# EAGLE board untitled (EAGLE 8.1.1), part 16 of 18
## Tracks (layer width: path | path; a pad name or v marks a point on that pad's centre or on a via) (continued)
S$16206 (continued)
  Bottom 0: 76.33,152.19 76.33,151.84
S$16207
  Bottom 0: 76.33,151.84 76.42,151.51
S$16208
  Bottom 0: 76.42,151.51 76.48,151.4
S$16209
  Bottom 0: 76.48,151.4 73.88,148.81
S$16210
  Bottom 0: 73.88,148.81 73.84,148.75
S$16211
  Bottom 0: 73.84,148.75 73.8,148.69
S$16212
  Bottom 0: 73.8,148.69 73.78,148.63
S$16213
  Bottom 0: 73.78,148.63 73.76,148.56
S$16214
  Bottom 0: 73.76,148.56 73.76,148.49
S$16215
  Bottom 0: 73.76,148.49 73.76,148.43
S$16216
  Bottom 0: 73.76,148.43 71.89,146.57
S$16217
  Bottom 0: 71.89,146.57 42.96,146.57
S$16218
  Bottom 0: 42.96,146.57 42.89,146.57
S$16219
  Bottom 0: 42.89,146.57 42.82,146.55
S$16220
  Bottom 0: 42.82,146.55 42.76,146.53
S$16221
  Bottom 0: 42.76,146.53 42.7,146.49
S$16222
  Bottom 0: 42.7,146.49 42.64,146.44
S$16223
  Bottom 0: 42.64,146.44 40.87,144.67
S$16224
  Bottom 0: 71.46,148.09 71.81,148.15
S$16225
  Bottom 0: 71.81,148.15 72.12,148.3
S$16226
  Bottom 0: 72.12,148.3 72.39,148.52
S$16227
  Bottom 0: 72.39,148.52 72.6,148.81
S$16228
  Bottom 0: 72.6,148.81 72.72,149.13
S$16229
  Bottom 0: 72.72,149.13 72.77,149.48
S$16230
  Bottom 0: 72.77,149.48 72.72,149.82
S$16231
  Bottom 0: 72.72,149.82 72.6,150.15
S$16232
  Bottom 0: 72.6,150.15 72.39,150.43
S$16233
  Bottom 0: 72.39,150.43 72.12,150.66
S$16234
  Bottom 0: 72.12,150.66 71.81,150.81
S$16235
  Bottom 0: 71.81,150.81 71.46,150.87
S$16236
  Bottom 0: 71.46,150.87 71.11,150.85
S$16237
  Bottom 0: 71.11,150.85 70.78,150.74
S$16238
  Bottom 0: 70.78,150.74 70.75,150.72
S$16239
  Bottom 0: 70.75,150.72 70.17,151.3
S$16240
  Bottom 0: 70.17,151.3 70.12,151.34
S$16241
  Bottom 0: 70.12,151.34 70.06,151.38
S$16242
  Bottom 0: 70.06,151.38 70,151.4
S$16243
  Bottom 0: 70,151.4 69.94,151.42
S$16244
  Bottom 0: 69.94,151.42 69.86,151.43
S$16245
  Bottom 0: 69.86,151.43 65.29,151.43
S$16246
  Bottom 0: 65.29,151.43 65.22,151.56
S$16247
  Bottom 0: 65.22,151.56 65.02,151.78
S$16248
  Bottom 0: 65.02,151.78 64.76,151.93
S$16249
  Bottom 0: 64.76,151.93 64.46,151.99
S$16250
  Bottom 0: 64.46,151.99 64.16,151.97
S$16251
  Bottom 0: 64.16,151.97 63.88,151.86
S$16252
  Bottom 0: 63.88,151.86 63.64,151.67
S$16253
  Bottom 0: 63.64,151.67 63.47,151.43
S$16254
  Bottom 0: 63.47,151.43 63.38,151.13
S$16255
  Bottom 0: 63.38,151.13 63.38,150.83
S$16256
  Bottom 0: 63.38,150.83 63.47,150.54
S$16257
  Bottom 0: 63.47,150.54 63.64,150.29
S$16258
  Bottom 0: 63.64,150.29 63.88,150.1
S$16259
  Bottom 0: 63.88,150.1 64.16,149.99
S$16260
  Bottom 0: 64.16,149.99 64.46,149.97
S$16261
  Bottom 0: 64.46,149.97 64.76,150.04
S$16262
  Bottom 0: 64.76,150.04 65.02,150.19
S$16263
  Bottom 0: 65.02,150.19 65.22,150.41
S$16264
  Bottom 0: 65.22,150.41 65.29,150.54
S$16265
  Bottom 0: 65.29,150.54 69.68,150.54
S$16266
  Bottom 0: 69.68,150.54 70.13,150.09
S$16267
  Bottom 0: 70.13,150.09 70.07,149.99
S$16268
  Bottom 0: 70.07,149.99 69.98,149.65
S$16269
  Bottom 0: 69.98,149.65 69.98,149.3
S$16270
  Bottom 0: 69.98,149.3 70.07,148.97
S$16271
  Bottom 0: 70.07,148.97 70.24,148.66
S$16272
  Bottom 0: 70.24,148.66 70.48,148.4
S$16273
  Bottom 0: 70.48,148.4 70.78,148.21
S$16274
  Bottom 0: 70.78,148.21 71.11,148.11
S$16275
  Bottom 0: 71.11,148.11 71.46,148.09
S$16276
  Bottom 0: 52.41,148.09 52.76,148.15
S$16277
  Bottom 0: 52.76,148.15 53.07,148.3
S$16278
  Bottom 0: 53.07,148.3 53.34,148.52
S$16279
  Bottom 0: 53.34,148.52 53.55,148.81
S$16280
  Bottom 0: 53.55,148.81 53.67,149.13
S$16281
  Bottom 0: 53.67,149.13 53.72,149.48
S$16282
  Bottom 0: 53.72,149.48 53.67,149.82
S$16283
  Bottom 0: 53.67,149.82 53.55,150.15
S$16284
  Bottom 0: 53.55,150.15 53.34,150.43
S$16285
  Bottom 0: 53.34,150.43 53.07,150.66
S$16286
  Bottom 0: 53.07,150.66 52.76,150.81
S$16287
  Bottom 0: 52.76,150.81 52.41,150.87
S$16288
  Bottom 0: 52.41,150.87 52.06,150.85
S$16289
  Bottom 0: 52.06,150.85 51.73,150.74
S$16290
  Bottom 0: 51.73,150.74 51.7,150.73
S$16291
  Bottom 0: 51.7,150.73 51.13,151.3
S$16292
  Bottom 0: 51.13,151.3 51.08,151.34
S$16293
  Bottom 0: 51.08,151.34 51.02,151.38
S$16294
  Bottom 0: 51.02,151.38 50.96,151.4
S$16295
  Bottom 0: 50.96,151.4 50.89,151.42
S$16296
  Bottom 0: 50.89,151.42 50.82,151.43
S$16297
  Bottom 0: 50.82,151.43 46.24,151.43
S$16298
  Bottom 0: 46.24,151.43 46.17,151.56
S$16299
  Bottom 0: 46.17,151.56 45.97,151.78
S$16300
  Bottom 0: 45.97,151.78 45.71,151.93
S$16301
  Bottom 0: 45.71,151.93 45.41,151.99
S$16302
  Bottom 0: 45.41,151.99 45.11,151.97
S$16303
  Bottom 0: 45.11,151.97 44.83,151.86
S$16304
  Bottom 0: 44.83,151.86 44.59,151.67
S$16305
  Bottom 0: 44.59,151.67 44.42,151.43
S$16306
  Bottom 0: 44.42,151.43 44.33,151.13
S$16307
  Bottom 0: 44.33,151.13 44.33,150.83
S$16308
  Bottom 0: 44.33,150.83 44.42,150.54
S$16309
  Bottom 0: 44.42,150.54 44.59,150.29
S$16310
  Bottom 0: 44.59,150.29 44.83,150.1
S$16311
  Bottom 0: 44.83,150.1 45.11,149.99
S$16312
  Bottom 0: 45.11,149.99 45.41,149.97
S$16313
  Bottom 0: 45.41,149.97 45.71,150.04
S$16314
  Bottom 0: 45.71,150.04 45.97,150.19
S$16315
  Bottom 0: 45.97,150.19 46.17,150.41
S$16316
  Bottom 0: 46.17,150.41 46.24,150.54
S$16317
  Bottom 0: 46.24,150.54 50.63,150.54
S$16318
  Bottom 0: 50.63,150.54 51.08,150.09
S$16319
  Bottom 0: 51.08,150.09 51.02,149.99
S$16320
  Bottom 0: 51.02,149.99 50.94,149.65
S$16321
  Bottom 0: 50.94,149.65 50.94,149.3
S$16322
  Bottom 0: 50.94,149.3 51.02,148.97
S$16323
  Bottom 0: 51.02,148.97 51.19,148.66
S$16324
  Bottom 0: 51.19,148.66 51.44,148.4
S$16325
  Bottom 0: 51.44,148.4 51.73,148.21
S$16326
  Bottom 0: 51.73,148.21 52.06,148.11
S$16327
  Bottom 0: 52.06,148.11 52.41,148.09
S$16328
  Bottom 0: 58.76,150.63 59.11,150.69
S$16329
  Bottom 0: 59.11,150.69 59.42,150.84
S$16330
  Bottom 0: 59.42,150.84 59.69,151.06
S$16331
  Bottom 0: 59.69,151.06 59.9,151.35
S$16332
  Bottom 0: 59.9,151.35 60.02,151.67
S$16333
  Bottom 0: 60.02,151.67 60.07,152.02
S$16334
  Bottom 0: 60.07,152.02 60.02,152.36
S$16335
  Bottom 0: 60.02,152.36 59.9,152.69
S$16336
  Bottom 0: 59.9,152.69 59.69,152.97
S$16337
  Bottom 0: 59.69,152.97 59.42,153.2
S$16338
  Bottom 0: 59.42,153.2 59.11,153.35
S$16339
  Bottom 0: 59.11,153.35 58.76,153.41
S$16340
  Bottom 0: 58.76,153.41 58.41,153.39
S$16341
  Bottom 0: 58.41,153.39 58.08,153.28
S$16342
  Bottom 0: 58.08,153.28 57.78,153.1
S$16343
  Bottom 0: 57.78,153.1 57.54,152.84
S$16344
  Bottom 0: 57.54,152.84 57.37,152.53
S$16345
  Bottom 0: 57.37,152.53 57.28,152.19
S$16346
  Bottom 0: 57.28,152.19 57.28,151.84
S$16347
  Bottom 0: 57.28,151.84 57.37,151.51
S$16348
  Bottom 0: 57.37,151.51 57.54,151.2
S$16349
  Bottom 0: 57.54,151.2 57.78,150.94
S$16350
  Bottom 0: 57.78,150.94 58.08,150.75
S$16351
  Bottom 0: 58.08,150.75 58.41,150.65
S$16352
  Bottom 0: 58.41,150.65 58.76,150.63
S$16353
  Bottom 0: 35.81,152.27 36.26,152.32
S$16354
  Bottom 0: 36.26,152.32 36.69,152.45
S$16355
  Bottom 0: 36.69,152.45 37.08,152.66
S$16356
  Bottom 0: 37.08,152.66 37.43,152.94
S$16357
  Bottom 0: 37.43,152.94 37.71,153.29
S$16358
  Bottom 0: 37.71,153.29 37.93,153.68
S$16359
  Bottom 0: 37.93,153.68 38.05,154.11
S$16360
  Bottom 0: 38.05,154.11 38.1,154.56
S$16361
  Bottom 0: 38.1,154.56 38.05,155.01
S$16362
  Bottom 0: 38.05,155.01 37.93,155.43
S$16363
  Bottom 0: 37.93,155.43 37.71,155.83
S$16364
  Bottom 0: 37.71,155.83 37.43,156.17
S$16365
  Bottom 0: 37.43,156.17 37.08,156.46
S$16366
  Bottom 0: 37.08,156.46 36.69,156.67
S$16367
  Bottom 0: 36.69,156.67 36.26,156.8
S$16368
  Bottom 0: 36.26,156.8 35.81,156.84
S$16369
  Bottom 0: 35.81,156.84 35.37,156.8
S$16370
  Bottom 0: 35.37,156.8 34.94,156.67
S$16371
  Bottom 0: 34.94,156.67 34.54,156.46
S$16372
  Bottom 0: 34.54,156.46 34.2,156.17
S$16373
  Bottom 0: 34.2,156.17 33.91,155.83
S$16374
  Bottom 0: 33.91,155.83 33.7,155.43
S$16375
  Bottom 0: 33.7,155.43 33.57,155.01
S$16376
  Bottom 0: 33.57,155.01 33.53,154.56
S$16377
  Bottom 0: 33.53,154.56 33.57,154.11
S$16378
  Bottom 0: 33.57,154.11 33.7,153.68
S$16379
  Bottom 0: 33.7,153.68 33.91,153.29
S$16380
  Bottom 0: 33.91,153.29 34.2,152.94
S$16381
  Bottom 0: 34.2,152.94 34.54,152.66
S$16382
  Bottom 0: 34.54,152.66 34.94,152.45
S$16383
  Bottom 0: 34.94,152.45 35.37,152.32
S$16384
  Bottom 0: 35.37,152.32 35.81,152.27
S$16385
  Bottom 0: 315.71,144.69 309.34,151.06
S$16386
  Bottom 0: 309.34,151.06 309.34,156.73
S$16387
  Bottom 0: 309.34,156.73 315.71,150.37
S$16388
  Bottom 0: 315.71,150.37 315.71,144.69
S$16389
  Bottom 0: 313.57,148.07 313.88,148.13
S$16390
  Bottom 0: 313.88,148.13 313.99,148.09
S$16391
  Bottom 0: 313.99,148.09 314.33,148.07
S$16392
  Bottom 0: 314.33,148.07 314.68,148.13
S$16393
  Bottom 0: 314.68,148.13 315,148.28
S$16394
  Bottom 0: 315,148.28 315.26,148.51
S$16395
  Bottom 0: 315.26,148.51 315.47,148.79
S$16396
  Bottom 0: 315.47,148.79 315.6,149.12
S$16397
  Bottom 0: 315.6,149.12 315.65,149.46
S$16398
  Bottom 0: 315.65,149.46 315.6,149.81
S$16399
  Bottom 0: 315.6,149.81 315.47,150.13
S$16400
  Bottom 0: 315.47,150.13 315.26,150.42
S$16401
  Bottom 0: 315.26,150.42 315,150.64
S$16402
  Bottom 0: 315,150.64 314.68,150.79
S$16403
  Bottom 0: 314.68,150.79 314.33,150.85
S$16404
  Bottom 0: 314.33,150.85 313.99,150.84
S$16405
  Bottom 0: 313.99,150.84 313.88,150.8
S$16406
  Bottom 0: 313.88,150.8 313.57,150.85
S$16407
  Bottom 0: 313.57,150.85 313.22,150.84
S$16408
  Bottom 0: 313.22,150.84 312.89,150.73
S$16409
  Bottom 0: 312.89,150.73 312.6,150.54
S$16410
  Bottom 0: 312.6,150.54 312.36,150.29
S$16411
  Bottom 0: 312.36,150.29 312.19,149.98
S$16412
  Bottom 0: 312.19,149.98 312.1,149.64
S$16413
  Bottom 0: 312.1,149.64 312.1,149.29
S$16414
  Bottom 0: 312.1,149.29 312.19,148.95
S$16415
  Bottom 0: 312.19,148.95 312.36,148.64
S$16416
  Bottom 0: 312.36,148.64 312.6,148.39
S$16417
  Bottom 0: 312.6,148.39 312.89,148.2
S$16418
  Bottom 0: 312.89,148.2 313.22,148.09
S$16419
  Bottom 0: 313.22,148.09 313.57,148.07
S$16420
  Bottom 0: 149.44,144.78 149.44,146.12
S$16421
  Bottom 0: 149.44,146.12 153.95,150.63
S$16422
  Bottom 0: 153.95,150.63 154.01,150.63
S$16423
  Bottom 0: 154.01,150.63 154.36,150.69
S$16424
  Bottom 0: 154.36,150.69 154.67,150.84
S$16425
  Bottom 0: 154.67,150.84 154.94,151.06
S$16426
  Bottom 0: 154.94,151.06 155.15,151.35
S$16427
  Bottom 0: 155.15,151.35 155.28,151.67
S$16428
  Bottom 0: 155.28,151.67 155.32,152.02
S$16429
  Bottom 0: 155.32,152.02 155.28,152.36
S$16430
  Bottom 0: 155.28,152.36 155.15,152.69
S$16431
  Bottom 0: 155.15,152.69 154.94,152.97
S$16432
  Bottom 0: 154.94,152.97 154.68,153.19
S$16433
  Bottom 0: 154.68,153.19 154.68,158.72
S$16434
  Bottom 0: 154.68,158.72 156.88,156.53
S$16435
  Bottom 0: 156.88,156.53 156.88,153.11
S$16436
  Bottom 0: 156.88,153.11 156.74,152.96
S$16437
  Bottom 0: 156.74,152.96 156.65,152.72
S$16438
  Bottom 0: 156.65,152.72 156.65,152.47
S$16439
  Bottom 0: 156.65,152.47 156.74,152.24
S$16440
  Bottom 0: 156.74,152.24 156.81,152.16
S$16441
  Bottom 0: 156.81,152.16 156.76,152.12
S$16442
  Bottom 0: 156.76,152.12 149.46,144.82
S$16443
  Bottom 0: 149.46,144.82 149.44,144.78
S$16444
  Bottom 0: 316.4,150.93 309.9,157.42
S$16445
  Bottom 0: 309.9,157.42 309.9,158.28
S$16446
  Bottom 0: 309.9,158.28 309.89,158.35
S$16447
  Bottom 0: 309.89,158.35 309.88,158.42
S$16448
  Bottom 0: 309.88,158.42 309.86,158.48
S$16449
  Bottom 0: 309.86,158.48 309.81,158.54
S$16450
  Bottom 0: 309.81,158.54 309.77,158.6
S$16451
  Bottom 0: 309.77,158.6 308.42,159.95
S$16452
  Bottom 0: 308.42,159.95 308.93,159.95
S$16453
  Bottom 0: 308.93,159.95 310.94,157.95
S$16454
  Bottom 0: 310.94,157.95 310.99,157.91
S$16455
  Bottom 0: 310.99,157.91 311.05,157.87
S$16456
  Bottom 0: 311.05,157.87 311.11,157.84
S$16457
  Bottom 0: 311.11,157.84 311.18,157.82
S$16458
  Bottom 0: 311.18,157.82 311.25,157.82
S$16459
  Bottom 0: 311.25,157.82 318.62,157.82
S$16460
  Bottom 0: 318.62,157.82 318.69,157.82
S$16461
  Bottom 0: 318.69,157.82 318.76,157.84
S$16462
  Bottom 0: 318.76,157.84 318.82,157.87
S$16463
  Bottom 0: 318.82,157.87 318.88,157.91
S$16464
  Bottom 0: 318.88,157.91 318.94,157.95
S$16465
  Bottom 0: 318.94,157.95 319.65,158.66
S$16466
  Bottom 0: 319.65,158.66 319.69,158.71
S$16467
  Bottom 0: 319.69,158.71 319.73,158.78
S$16468
  Bottom 0: 319.73,158.78 319.76,158.84
S$16469
  Bottom 0: 319.76,158.84 319.77,158.9
S$16470
  Bottom 0: 319.77,158.9 319.78,158.97
S$16471
  Bottom 0: 319.78,158.97 319.78,162.09
S$16472
  Bottom 0: 319.78,162.09 319.95,161.92
S$16473
  Bottom 0: 319.95,161.92 320.24,161.77
S$16474
  Bottom 0: 320.24,161.77 320.56,161.71
S$16475
  Bottom 0: 320.56,161.71 320.89,161.73
S$16476
  Bottom 0: 320.89,161.73 321.19,161.83
S$16477
  Bottom 0: 321.19,161.83 321.46,162.02
S$16478
  Bottom 0: 321.46,162.02 321.67,162.28
S$16479
  Bottom 0: 321.67,162.28 321.73,162.43
S$16480
  Bottom 0: 321.73,162.43 321.73,156.69
S$16481
  Bottom 0: 321.73,156.69 318.97,153.92
S$16482
  Bottom 0: 318.97,153.92 319.02,154.1
S$16483
  Bottom 0: 319.02,154.1 319.07,154.54
S$16484
  Bottom 0: 319.07,154.54 319.02,154.99
S$16485
  Bottom 0: 319.02,154.99 318.9,155.42
S$16486
  Bottom 0: 318.9,155.42 318.68,155.81
S$16487
  Bottom 0: 318.68,155.81 318.4,156.16
S$16488
  Bottom 0: 318.4,156.16 318.05,156.44
S$16489
  Bottom 0: 318.05,156.44 317.65,156.66
S$16490
  Bottom 0: 317.65,156.66 317.23,156.78
S$16491
  Bottom 0: 317.23,156.78 316.78,156.83
S$16492
  Bottom 0: 316.78,156.83 316.4,156.79
S$16493
  Bottom 0: 316.4,156.79 316.02,156.83
S$16494
  Bottom 0: 316.02,156.83 315.57,156.78
S$16495
  Bottom 0: 315.57,156.78 315.15,156.66
S$16496
  Bottom 0: 315.15,156.66 314.75,156.44
S$16497
  Bottom 0: 314.75,156.44 314.41,156.16
S$16498
  Bottom 0: 314.41,156.16 314.12,155.81
S$16499
  Bottom 0: 314.12,155.81 313.91,155.42
S$16500
  Bottom 0: 313.91,155.42 313.78,154.99
S$16501
  Bottom 0: 313.78,154.99 313.74,154.54
S$16502
  Bottom 0: 313.74,154.54 313.78,154.1
S$16503
  Bottom 0: 313.78,154.1 313.91,153.67
S$16504
  Bottom 0: 313.91,153.67 314.12,153.27
S$16505
  Bottom 0: 314.12,153.27 314.41,152.93
S$16506
  Bottom 0: 314.41,152.93 314.75,152.64
S$16507
  Bottom 0: 314.75,152.64 315.15,152.43
S$16508
  Bottom 0: 315.15,152.43 315.57,152.3
S$16509
  Bottom 0: 315.57,152.3 316.02,152.26
S$16510
  Bottom 0: 316.02,152.26 316.4,152.3
S$16511
  Bottom 0: 316.4,152.3 316.78,152.26
S$16512
  Bottom 0: 316.78,152.26 317.23,152.3
S$16513
  Bottom 0: 317.23,152.3 317.4,152.35
S$16514
  Bottom 0: 317.4,152.35 316.53,151.48
S$16515
  Bottom 0: 316.53,151.48 316.49,151.43
S$16516
  Bottom 0: 316.49,151.43 316.45,151.37
S$16517
  Bottom 0: 316.45,151.37 316.42,151.31
S$16518
  Bottom 0: 316.42,151.31 316.41,151.24
S$16519
  Bottom 0: 316.41,151.24 316.4,151.17
S$16520
  Bottom 0: 316.4,151.17 316.4,150.93
S$16521
  Bottom 0: 254.44,152.46 254.52,152.58
S$16522
  Bottom 0: 254.52,152.58 254.56,152.83
S$16523
  Bottom 0: 254.56,152.83 254.52,153.08
S$16524
  Bottom 0: 254.52,153.08 254.39,153.29
S$16525
  Bottom 0: 254.39,153.29 254.18,153.45
S$16526
  Bottom 0: 254.18,153.45 253.94,153.51
S$16527
  Bottom 0: 253.94,153.51 253.84,153.5
S$16528
  Bottom 0: 253.84,153.5 248.84,158.5
S$16529
  Bottom 0: 248.84,158.5 248.79,158.54
S$16530
  Bottom 0: 248.79,158.54 248.73,158.57
S$16531
  Bottom 0: 248.73,158.57 248.67,158.6
S$16532
  Bottom 0: 248.67,158.6 248.6,158.62
S$16533
  Bottom 0: 248.6,158.62 248.53,158.62
S$16534
  Bottom 0: 248.53,158.62 247.15,158.62
S$16535
  Bottom 0: 247.15,158.62 247.38,158.78
S$16536
  Bottom 0: 247.38,158.78 247.59,159.02
S$16537
  Bottom 0: 247.59,159.02 247.73,159.32
S$16538
  Bottom 0: 247.73,159.32 247.78,159.64
S$16539
  Bottom 0: 247.78,159.64 247.73,159.96
S$16540
  Bottom 0: 247.73,159.96 247.59,160.26
S$16541
  Bottom 0: 247.59,160.26 247.38,160.5
S$16542
  Bottom 0: 247.38,160.5 247.1,160.68
S$16543
  Bottom 0: 247.1,160.68 246.8,160.77
S$16544
  Bottom 0: 246.8,160.77 246.47,160.77
S$16545
  Bottom 0: 246.47,160.77 246.16,160.68
S$16546
  Bottom 0: 246.16,160.68 245.89,160.5
S$16547
  Bottom 0: 245.89,160.5 245.81,160.41
S$16548
  Bottom 0: 245.81,160.41 245.81,161.9
S$16549
  Bottom 0: 245.81,161.9 245.8,161.98
S$16550
  Bottom 0: 245.8,161.98 245.79,162.04
S$16551
  Bottom 0: 245.79,162.04 245.76,162.1
S$16552
  Bottom 0: 245.76,162.1 245.72,162.16
S$16553
  Bottom 0: 245.72,162.16 245.68,162.22
S$16554
  Bottom 0: 245.68,162.22 238.52,169.38
S$16555
  Bottom 0: 238.52,169.38 238.52,170.26
S$16556
  Bottom 0: 238.52,170.26 238.52,170.25
S$16557
  Bottom 0: 238.52,170.25 238.76,169.99
S$16558
  Bottom 0: 238.76,169.99 239.06,169.8
S$16559
  Bottom 0: 239.06,169.8 239.38,169.7
S$16560
  Bottom 0: 239.38,169.7 239.72,169.68
S$16561
  Bottom 0: 239.72,169.68 248.45,160.94
S$16562
  Bottom 0: 248.45,160.94 248.5,160.9
S$16563
  Bottom 0: 248.5,160.9 248.56,160.86
S$16564
  Bottom 0: 248.56,160.86 248.62,160.84
S$16565
  Bottom 0: 248.62,160.84 248.69,160.82
S$16566
  Bottom 0: 248.69,160.82 248.76,160.82
S$16567
  Bottom 0: 248.76,160.82 250.71,160.82
S$16568
  Bottom 0: 250.71,160.82 254.9,156.63
S$16569
  Bottom 0: 254.9,156.63 254.96,156.58
S$16570
  Bottom 0: 254.96,156.58 255.01,156.54
S$16571
  Bottom 0: 255.01,156.54 255.08,156.51
S$16572
  Bottom 0: 255.08,156.51 255.14,156.5
S$16573
  Bottom 0: 255.14,156.5 255.21,156.49
S$16574
  Bottom 0: 255.21,156.49 258.72,156.49
S$16575
  Bottom 0: 258.72,156.49 258.79,156.5
S$16576
  Bottom 0: 258.79,156.5 258.85,156.51
S$16577
  Bottom 0: 258.85,156.51 258.92,156.54
S$16578
  Bottom 0: 258.92,156.54 258.98,156.58
S$16579
  Bottom 0: 258.98,156.58 259.03,156.62
S$16580
  Bottom 0: 259.03,156.62 259.38,156.97
S$16581
  Bottom 0: 259.38,156.97 260.19,156.97
S$16582
  Bottom 0: 260.19,156.97 260.12,156.92
S$16583
  Bottom 0: 260.12,156.92 259.95,156.66
S$16584
  Bottom 0: 259.95,156.66 259.86,156.38
S$16585
  Bottom 0: 259.86,156.38 259.86,156.07
S$16586
  Bottom 0: 259.86,156.07 259.95,155.78
S$16587
  Bottom 0: 259.95,155.78 260.12,155.53
S$16588
  Bottom 0: 260.12,155.53 260.36,155.35
S$16589
  Bottom 0: 260.36,155.35 260.64,155.24
S$16590
  Bottom 0: 260.64,155.24 260.94,155.21
S$16591
  Bottom 0: 260.94,155.21 261.24,155.28
S$16592
  Bottom 0: 261.24,155.28 261.5,155.43
S$16593
  Bottom 0: 261.5,155.43 261.7,155.65
S$16594
  Bottom 0: 261.7,155.65 261.84,155.93
S$16595
  Bottom 0: 261.84,155.93 261.88,156.22
S$16596
  Bottom 0: 261.88,156.22 261.84,156.53
S$16597
  Bottom 0: 261.84,156.53 261.7,156.8
S$16598
  Bottom 0: 261.7,156.8 261.55,156.97
S$16599
  Bottom 0: 261.55,156.97 264.51,156.97
S$16600
  Bottom 0: 264.51,156.97 264.73,156.75
S$16601
  Bottom 0: 264.73,156.75 264.79,156.71
S$16602
  Bottom 0: 264.79,156.71 264.85,156.66
S$16603
  Bottom 0: 264.85,156.66 264.91,156.64
S$16604
  Bottom 0: 264.91,156.64 264.97,156.63
S$16605
  Bottom 0: 264.97,156.63 265.04,156.62
S$16606
  Bottom 0: 265.04,156.62 268.2,156.62
S$16607
  Bottom 0: 268.2,156.62 267.9,156.46
S$16608
  Bottom 0: 267.9,156.46 267.56,156.17
S$16609
  Bottom 0: 267.56,156.17 267.27,155.83
S$16610
  Bottom 0: 267.27,155.83 267.06,155.43
S$16611
  Bottom 0: 267.06,155.43 266.93,155.01
S$16612
  Bottom 0: 266.93,155.01 266.89,154.56
S$16613
  Bottom 0: 266.89,154.56 266.93,154.11
S$16614
  Bottom 0: 266.93,154.11 267.06,153.68
S$16615
  Bottom 0: 267.06,153.68 267.27,153.29
S$16616
  Bottom 0: 267.27,153.29 267.56,152.94
S$16617
  Bottom 0: 267.56,152.94 267.9,152.66
S$16618
  Bottom 0: 267.9,152.66 268.27,152.46
S$16619
  Bottom 0: 268.27,152.46 254.44,152.46
S$16620
  Bottom 0: 253.8,155.21 254.1,155.28
S$16621
  Bottom 0: 254.1,155.28 254.36,155.43
S$16622
  Bottom 0: 254.36,155.43 254.56,155.65
S$16623
  Bottom 0: 254.56,155.65 254.7,155.93
S$16624
  Bottom 0: 254.7,155.93 254.74,156.22
S$16625
  Bottom 0: 254.74,156.22 254.7,156.53
S$16626
  Bottom 0: 254.7,156.53 254.56,156.8
S$16627
  Bottom 0: 254.56,156.8 254.36,157.02
S$16628
  Bottom 0: 254.36,157.02 254.1,157.17
S$16629
  Bottom 0: 254.1,157.17 253.8,157.24
S$16630
  Bottom 0: 253.8,157.24 253.5,157.22
S$16631
  Bottom 0: 253.5,157.22 253.22,157.1
S$16632
  Bottom 0: 253.22,157.1 252.98,156.92
S$16633
  Bottom 0: 252.98,156.92 252.81,156.66
S$16634
  Bottom 0: 252.81,156.66 252.72,156.38
S$16635
  Bottom 0: 252.72,156.38 252.72,156.07
S$16636
  Bottom 0: 252.72,156.07 252.81,155.78
S$16637
  Bottom 0: 252.81,155.78 252.98,155.53
S$16638
  Bottom 0: 252.98,155.53 253.22,155.35
S$16639
  Bottom 0: 253.22,155.35 253.5,155.24
S$16640
  Bottom 0: 253.5,155.24 253.8,155.21
S$16641
  Bottom 0: 255.4,157.38 253.45,159.33
S$16642
  Bottom 0: 253.45,159.33 253.73,159.34
S$16643
  Bottom 0: 253.73,159.34 254.04,159.45
S$16644
  Bottom 0: 254.04,159.45 254.3,159.64
S$16645
  Bottom 0: 254.3,159.64 254.51,159.89
S$16646
  Bottom 0: 254.51,159.89 254.63,160.19
S$16647
  Bottom 0: 254.63,160.19 254.68,160.51
S$16648
  Bottom 0: 254.68,160.51 254.63,160.83
S$16649
  Bottom 0: 254.63,160.83 254.51,161.13
S$16650
  Bottom 0: 254.51,161.13 254.3,161.39
S$16651
  Bottom 0: 254.3,161.39 254.04,161.57
S$16652
  Bottom 0: 254.04,161.57 253.73,161.68
S$16653
  Bottom 0: 253.73,161.68 253.41,161.7
S$16654
  Bottom 0: 253.41,161.7 253.16,161.65
S$16655
  Bottom 0: 253.16,161.65 251.51,163.3
S$16656
  Bottom 0: 251.51,163.3 251.44,163.36
S$16657
  Bottom 0: 251.44,163.36 251.37,163.4
S$16658
  Bottom 0: 251.37,163.4 251.29,163.44
S$16659
  Bottom 0: 251.29,163.44 251.2,163.46
S$16660
  Bottom 0: 251.2,163.46 251.11,163.46
S$16661
  Bottom 0: 251.11,163.46 250.24,163.46
S$16662
  Bottom 0: 250.24,163.46 250.22,163.51
S$16663
  Bottom 0: 250.22,163.51 250.01,163.77
S$16664
  Bottom 0: 250.01,163.77 249.75,163.96
S$16665
  Bottom 0: 249.75,163.96 249.44,164.06
S$16666
  Bottom 0: 249.44,164.06 249.12,164.08
S$16667
  Bottom 0: 249.12,164.08 248.8,164.02
S$16668
  Bottom 0: 248.8,164.02 248.51,163.87
S$16669
  Bottom 0: 248.51,163.87 248.28,163.65
S$16670
  Bottom 0: 248.28,163.65 248.1,163.37
S$16671
  Bottom 0: 248.1,163.37 248.02,163.06
S$16672
  Bottom 0: 248.02,163.06 248.02,162.73
S$16673
  Bottom 0: 248.02,162.73 248.05,162.6
S$16674
  Bottom 0: 248.05,162.6 240.59,170.06
S$16675
  Bottom 0: 240.59,170.06 240.66,170.11
S$16676
  Bottom 0: 240.66,170.11 240.87,170.4
S$16677
  Bottom 0: 240.87,170.4 241,170.72
S$16678
  Bottom 0: 241,170.72 241.05,171.07
S$16679
  Bottom 0: 241.05,171.07 241,171.41
S$16680
  Bottom 0: 241,171.41 240.87,171.74
S$16681
  Bottom 0: 240.87,171.74 240.66,172.02
S$16682
  Bottom 0: 240.66,172.02 240.4,172.25
S$16683
  Bottom 0: 240.4,172.25 240.08,172.4
S$16684
  Bottom 0: 240.08,172.4 239.73,172.46
S$16685
  Bottom 0: 239.73,172.46 239.42,172.44
S$16686
  Bottom 0: 239.42,172.44 243.74,176.76
S$16687
  Bottom 0: 243.74,176.76 243.97,176.67
S$16688
  Bottom 0: 243.97,176.67 244.28,176.65
S$16689
  Bottom 0: 244.28,176.65 244.57,176.71
S$16690
  Bottom 0: 244.57,176.71 244.84,176.87
S$16691
  Bottom 0: 244.84,176.87 245.04,177.08
S$16692
  Bottom 0: 245.04,177.08 245.17,177.36
S$16693
  Bottom 0: 245.17,177.36 245.22,177.66
S$16694
  Bottom 0: 245.22,177.66 245.17,177.96
S$16695
  Bottom 0: 245.17,177.96 245.04,178.23
S$16696
  Bottom 0: 245.04,178.23 244.87,178.41
S$16697
  Bottom 0: 244.87,178.41 245.27,178.41
S$16698
  Bottom 0: 245.27,178.41 246.78,176.9
S$16699
  Bottom 0: 246.78,176.9 246.85,176.84
S$16700
  Bottom 0: 246.85,176.84 246.93,176.79
S$16701
  Bottom 0: 246.93,176.79 247.01,176.76
S$16702
  Bottom 0: 247.01,176.76 247.1,176.74
S$16703
  Bottom 0: 247.1,176.74 247.19,176.73
S$16704
  Bottom 0: 247.19,176.73 264.3,176.73
S$16705
  Bottom 0: 264.3,176.73 264.39,176.74
S$16706
  Bottom 0: 264.39,176.74 264.48,176.76
S$16707
  Bottom 0: 264.48,176.76 264.56,176.79
S$16708
  Bottom 0: 264.56,176.79 264.63,176.84
S$16709
  Bottom 0: 264.63,176.84 264.7,176.9
S$16710
  Bottom 0: 264.7,176.9 265.39,177.6
S$16711
  Bottom 0: 265.39,177.6 265.52,177.56
S$16712
  Bottom 0: 265.52,177.56 265.82,177.56
S$16713
  Bottom 0: 265.82,177.56 265.74,177.35
S$16714
  Bottom 0: 265.74,177.35 265.74,177.09
S$16715
  Bottom 0: 265.74,177.09 265.83,176.86
S$16716
  Bottom 0: 265.83,176.86 266,176.67
S$16717
  Bottom 0: 266,176.67 266.22,176.56
S$16718
  Bottom 0: 266.22,176.56 266.44,176.54
S$16719
  Bottom 0: 266.44,176.54 266.44,174.66
S$16720
  Bottom 0: 266.44,174.66 266.31,174.88
S$16721
  Bottom 0: 266.31,174.88 266.03,175.22
S$16722
  Bottom 0: 266.03,175.22 265.68,175.51
S$16723
  Bottom 0: 265.68,175.51 265.29,175.72
S$16724
  Bottom 0: 265.29,175.72 264.86,175.85
S$16725
  Bottom 0: 264.86,175.85 264.41,175.9
S$16726
  Bottom 0: 264.41,175.9 263.97,175.85
S$16727
  Bottom 0: 263.97,175.85 263.54,175.72
S$16728
  Bottom 0: 263.54,175.72 263.14,175.51
S$16729
  Bottom 0: 263.14,175.51 262.8,175.22
S$16730
  Bottom 0: 262.8,175.22 262.51,174.88
S$16731
  Bottom 0: 262.51,174.88 262.3,174.48
S$16732
  Bottom 0: 262.3,174.48 262.17,174.06
S$16733
  Bottom 0: 262.17,174.06 262.13,173.61
S$16734
  Bottom 0: 262.13,173.61 262.17,173.16
S$16735
  Bottom 0: 262.17,173.16 262.3,172.74
S$16736
  Bottom 0: 262.3,172.74 262.51,172.34
S$16737
  Bottom 0: 262.51,172.34 262.8,171.99
S$16738
  Bottom 0: 262.8,171.99 263.14,171.71
S$16739
  Bottom 0: 263.14,171.71 263.54,171.5
S$16740
  Bottom 0: 263.54,171.5 263.97,171.37
S$16741
  Bottom 0: 263.97,171.37 264.41,171.32
S$16742
  Bottom 0: 264.41,171.32 264.86,171.37
S$16743
  Bottom 0: 264.86,171.37 265.16,171.46
S$16744
  Bottom 0: 265.16,171.46 264.06,170.36
S$16745
  Bottom 0: 264.06,170.36 264.02,170.31
S$16746
  Bottom 0: 264.02,170.31 263.98,170.25
S$16747
  Bottom 0: 263.98,170.25 263.95,170.19
S$16748
  Bottom 0: 263.95,170.19 263.93,170.12
S$16749
  Bottom 0: 263.93,170.12 263.93,170.05
S$16750
  Bottom 0: 263.93,170.05 263.93,163.97
S$16751
  Bottom 0: 263.93,163.97 261.57,161.6
S$16752
  Bottom 0: 261.57,161.6 261.35,161.68
S$16753
  Bottom 0: 261.35,161.68 261.03,161.7
S$16754
  Bottom 0: 261.03,161.7 260.71,161.63
S$16755
  Bottom 0: 260.71,161.63 260.42,161.49
S$16756
  Bottom 0: 260.42,161.49 260.18,161.26
S$16757
  Bottom 0: 260.18,161.26 260.01,160.99
S$16758
  Bottom 0: 260.01,160.99 259.92,160.68
S$16759
  Bottom 0: 259.92,160.68 259.92,160.35
S$16760
  Bottom 0: 259.92,160.35 260.01,160.03
S$16761
  Bottom 0: 260.01,160.03 260.18,159.76
S$16762
  Bottom 0: 260.18,159.76 260.42,159.54
S$16763
  Bottom 0: 260.42,159.54 260.71,159.39
S$16764
  Bottom 0: 260.71,159.39 261.03,159.32
S$16765
  Bottom 0: 261.03,159.32 261.35,159.34
S$16766
  Bottom 0: 261.35,159.34 261.66,159.45
S$16767
  Bottom 0: 261.66,159.45 261.92,159.64
S$16768
  Bottom 0: 261.92,159.64 262.13,159.89
S$16769
  Bottom 0: 262.13,159.89 262.25,160.19
S$16770
  Bottom 0: 262.25,160.19 262.3,160.51
S$16771
  Bottom 0: 262.3,160.51 262.25,160.83
S$16772
  Bottom 0: 262.25,160.83 262.19,160.97
S$16773
  Bottom 0: 262.19,160.97 264.69,163.47
S$16774
  Bottom 0: 264.69,163.47 264.73,163.52
S$16775
  Bottom 0: 264.73,163.52 264.77,163.59
S$16776
  Bottom 0: 264.77,163.59 264.8,163.65
S$16777
  Bottom 0: 264.8,163.65 264.81,163.71
S$16778
  Bottom 0: 264.81,163.71 264.81,163.78
S$16779
  Bottom 0: 264.81,163.78 264.81,169.87
S$16780
  Bottom 0: 264.81,169.87 267.19,172.23
S$16781
  Bottom 0: 267.19,172.23 267.23,172.29
S$16782
  Bottom 0: 267.23,172.29 267.27,172.34
S$16783
  Bottom 0: 267.27,172.34 267.3,172.41
S$16784
  Bottom 0: 267.3,172.41 267.31,172.48
S$16785
  Bottom 0: 267.31,172.48 267.32,172.55
S$16786
  Bottom 0: 267.32,172.55 267.32,176.75
S$16787
  Bottom 0: 267.32,176.75 267.31,176.82
S$16788
  Bottom 0: 267.31,176.82 275.31,168.83
S$16789
  Bottom 0: 275.31,168.83 275.31,165.3
S$16790
  Bottom 0: 275.31,165.3 270.73,160.73
S$16791
  Bottom 0: 270.73,160.73 270.61,160.77
S$16792
  Bottom 0: 270.61,160.77 270.28,160.77
S$16793
  Bottom 0: 270.28,160.77 269.97,160.68
S$16794
  Bottom 0: 269.97,160.68 269.7,160.5
S$16795
  Bottom 0: 269.7,160.5 269.48,160.26
S$16796
  Bottom 0: 269.48,160.26 269.38,160.03
S$16797
  Bottom 0: 269.38,160.03 269.17,160.08
S$16798
  Bottom 0: 269.17,160.08 269.05,160.08
S$16799
  Bottom 0: 269.05,160.08 269.05,160.53
S$16800
  Bottom 0: 269.05,160.53 269.04,160.6
S$16801
  Bottom 0: 269.04,160.6 269,160.68
S$16802
  Bottom 0: 269,160.68 268.94,160.73
S$16803
  Bottom 0: 268.94,160.73 268.87,160.77
S$16804
  Bottom 0: 268.87,160.77 268.79,160.78
S$16805
  Bottom 0: 268.79,160.78 267.09,160.78
S$16806
  Bottom 0: 267.09,160.78 267.09,169.31
S$16807
  Bottom 0: 267.09,169.31 267.6,169.82
S$16808
  Bottom 0: 267.6,169.82 267.63,169.8
S$16809
  Bottom 0: 267.63,169.8 267.96,169.7
S$16810
  Bottom 0: 267.96,169.7 268.31,169.68
S$16811
  Bottom 0: 268.31,169.68 268.66,169.74
S$16812
  Bottom 0: 268.66,169.74 268.97,169.89
S$16813
  Bottom 0: 268.97,169.89 269.24,170.11
S$16814
  Bottom 0: 269.24,170.11 269.45,170.4
S$16815
  Bottom 0: 269.45,170.4 269.57,170.72
S$16816
  Bottom 0: 269.57,170.72 269.62,171.07
S$16817
  Bottom 0: 269.62,171.07 269.57,171.41
S$16818
  Bottom 0: 269.57,171.41 269.45,171.74
S$16819
  Bottom 0: 269.45,171.74 269.24,172.02
S$16820
  Bottom 0: 269.24,172.02 268.97,172.25
S$16821
  Bottom 0: 268.97,172.25 268.66,172.4
S$16822
  Bottom 0: 268.66,172.4 268.31,172.46
S$16823
  Bottom 0: 268.31,172.46 267.96,172.44
S$16824
  Bottom 0: 267.96,172.44 267.63,172.33
S$16825
  Bottom 0: 267.63,172.33 267.33,172.15
S$16826
  Bottom 0: 267.33,172.15 267.1,171.89
S$16827
  Bottom 0: 267.1,171.89 266.92,171.58
S$16828
  Bottom 0: 266.92,171.58 266.84,171.24
S$16829
  Bottom 0: 266.84,171.24 266.84,170.9
S$16830
  Bottom 0: 266.84,170.9 266.92,170.56
S$16831
  Bottom 0: 266.92,170.56 266.98,170.45
S$16832
  Bottom 0: 266.98,170.45 266.33,169.81
S$16833
  Bottom 0: 266.33,169.81 266.29,169.75
S$16834
  Bottom 0: 266.29,169.75 266.25,169.7
S$16835
  Bottom 0: 266.25,169.7 266.22,169.63
S$16836
  Bottom 0: 266.22,169.63 266.21,169.56
S$16837
  Bottom 0: 266.21,169.56 266.2,169.49
S$16838
  Bottom 0: 266.2,169.49 266.2,158.46
S$16839
  Bottom 0: 266.2,158.46 266.21,158.39
S$16840
  Bottom 0: 266.21,158.39 266.22,158.32
S$16841
  Bottom 0: 266.22,158.32 266.25,158.25
S$16842
  Bottom 0: 266.25,158.25 266.29,158.2
S$16843
  Bottom 0: 266.29,158.2 266.33,158.15
S$16844
  Bottom 0: 266.33,158.15 266.98,157.5
S$16845
  Bottom 0: 266.98,157.5 265.23,157.5
S$16846
  Bottom 0: 265.23,157.5 265.01,157.72
S$16847
  Bottom 0: 265.01,157.72 264.96,157.76
S$16848
  Bottom 0: 264.96,157.76 264.9,157.81
S$16849
  Bottom 0: 264.9,157.81 264.84,157.83
S$16850
  Bottom 0: 264.84,157.83 264.77,157.85
S$16851
  Bottom 0: 264.77,157.85 264.7,157.85
S$16852
  Bottom 0: 264.7,157.85 259.2,157.85
S$16853
  Bottom 0: 259.2,157.85 259.13,157.85
S$16854
  Bottom 0: 259.13,157.85 259.06,157.83
S$16855
  Bottom 0: 259.06,157.83 259,157.81
S$16856
  Bottom 0: 259,157.81 258.94,157.77
S$16857
  Bottom 0: 258.94,157.77 258.89,157.72
S$16858
  Bottom 0: 258.89,157.72 258.53,157.38
S$16859
  Bottom 0: 258.53,157.38 257.96,157.38
S$16860
  Bottom 0: 257.96,157.38 258.13,157.55
S$16861
  Bottom 0: 258.13,157.55 258.26,157.83
S$16862
  Bottom 0: 258.26,157.83 258.31,158.13
S$16863
  Bottom 0: 258.31,158.13 258.26,158.43
S$16864
  Bottom 0: 258.26,158.43 258.13,158.7
S$16865
  Bottom 0: 258.13,158.7 257.93,158.92
S$16866
  Bottom 0: 257.93,158.92 257.73,159.03
S$16867
  Bottom 0: 257.73,159.03 257.73,163.76
S$16868
  Bottom 0: 257.73,163.76 261.25,167.28
S$16869
  Bottom 0: 261.25,167.28 261.28,167.26
S$16870
  Bottom 0: 261.28,167.26 261.61,167.16
S$16871
  Bottom 0: 261.61,167.16 261.96,167.14
S$16872
  Bottom 0: 261.96,167.14 262.31,167.2
S$16873
  Bottom 0: 262.31,167.2 262.62,167.35
S$16874
  Bottom 0: 262.62,167.35 262.89,167.57
S$16875
  Bottom 0: 262.89,167.57 263.1,167.86
S$16876
  Bottom 0: 263.1,167.86 263.23,168.18
S$16877
  Bottom 0: 263.23,168.18 263.27,168.53
S$16878
  Bottom 0: 263.27,168.53 263.23,168.87
S$16879
  Bottom 0: 263.23,168.87 263.1,169.2
S$16880
  Bottom 0: 263.1,169.2 262.89,169.48
S$16881
  Bottom 0: 262.89,169.48 262.62,169.71
S$16882
  Bottom 0: 262.62,169.71 262.31,169.86
S$16883
  Bottom 0: 262.31,169.86 261.96,169.92
S$16884
  Bottom 0: 261.96,169.92 261.61,169.9
S$16885
  Bottom 0: 261.61,169.9 261.28,169.79
S$16886
  Bottom 0: 261.28,169.79 260.99,169.61
S$16887
  Bottom 0: 260.99,169.61 260.75,169.35
S$16888
  Bottom 0: 260.75,169.35 260.57,169.04
S$16889
  Bottom 0: 260.57,169.04 260.49,168.7
S$16890
  Bottom 0: 260.49,168.7 260.49,168.36
S$16891
  Bottom 0: 260.49,168.36 260.57,168.02
S$16892
  Bottom 0: 260.57,168.02 260.63,167.91
S$16893
  Bottom 0: 260.63,167.91 256.98,164.26
S$16894
  Bottom 0: 256.98,164.26 256.94,164.21
S$16895
  Bottom 0: 256.94,164.21 256.9,164.15
S$16896
  Bottom 0: 256.9,164.15 256.87,164.08
S$16897
  Bottom 0: 256.87,164.08 256.86,164.02
S$16898
  Bottom 0: 256.86,164.02 256.85,163.95
S$16899
  Bottom 0: 256.85,163.95 256.85,159.03
S$16900
  Bottom 0: 256.85,159.03 256.78,159.01
S$16901
  Bottom 0: 256.78,159.01 256.55,158.82
S$16902
  Bottom 0: 256.55,158.82 256.38,158.57
S$16903
  Bottom 0: 256.38,158.57 256.29,158.28
S$16904
  Bottom 0: 256.29,158.28 256.29,157.98
S$16905
  Bottom 0: 256.29,157.98 256.38,157.69
S$16906
  Bottom 0: 256.38,157.69 256.55,157.44
S$16907
  Bottom 0: 256.55,157.44 256.62,157.38
S$16908
  Bottom 0: 256.62,157.38 255.4,157.38
S$16909
  Bottom 0: 244.28,169.03 244.57,169.09
S$16910
  Bottom 0: 244.57,169.09 244.84,169.25
S$16911
  Bottom 0: 244.84,169.25 245.04,169.46
S$16912
  Bottom 0: 245.04,169.46 245.17,169.74
S$16913
  Bottom 0: 245.17,169.74 245.22,170.04
S$16914
  Bottom 0: 245.22,170.04 245.17,170.34
S$16915
  Bottom 0: 245.17,170.34 245.04,170.61
S$16916
  Bottom 0: 245.04,170.61 244.84,170.83
S$16917
  Bottom 0: 244.84,170.83 244.57,170.98
S$16918
  Bottom 0: 244.57,170.98 244.28,171.05
S$16919
  Bottom 0: 244.28,171.05 243.97,171.03
S$16920
  Bottom 0: 243.97,171.03 243.69,170.92
S$16921
  Bottom 0: 243.69,170.92 243.45,170.73
S$16922
  Bottom 0: 243.45,170.73 243.29,170.48
S$16923
  Bottom 0: 243.29,170.48 243.19,170.19
S$16924
  Bottom 0: 243.19,170.19 243.19,169.88
S$16925
  Bottom 0: 243.19,169.88 243.29,169.6
S$16926
  Bottom 0: 243.29,169.6 243.45,169.35
S$16927
  Bottom 0: 243.45,169.35 243.69,169.16
S$16928
  Bottom 0: 243.69,169.16 243.97,169.05
S$16929
  Bottom 0: 243.97,169.05 244.28,169.03
S$16930
  Bottom 0: 207.14,158.79 207.14,160.53
S$16931
  Bottom 0: 207.14,160.53 207.13,160.6
S$16932
  Bottom 0: 207.13,160.6 207.09,160.68
S$16933
  Bottom 0: 207.09,160.68 207.03,160.73
S$16934
  Bottom 0: 207.03,160.73 206.96,160.77
S$16935
  Bottom 0: 206.96,160.77 206.88,160.78
S$16936
  Bottom 0: 206.88,160.78 206.44,160.78
S$16937
  Bottom 0: 206.44,160.78 206.44,160.91
S$16938
  Bottom 0: 206.44,160.91 206.38,161.13
S$16939
  Bottom 0: 206.38,161.13 206.21,161.29
S$16940
  Bottom 0: 206.21,161.29 205.99,161.35
S$16941
  Bottom 0: 205.99,161.35 205.65,161.35
S$16942
  Bottom 0: 205.65,161.35 204.56,162.44
S$16943
  Bottom 0: 204.56,162.44 204.62,162.57
S$16944
  Bottom 0: 204.62,162.57 204.67,162.89
S$16945
  Bottom 0: 204.67,162.89 204.62,163.22
S$16946
  Bottom 0: 204.62,163.22 204.49,163.51
S$16947
  Bottom 0: 204.49,163.51 204.29,163.77
S$16948
  Bottom 0: 204.29,163.77 204.02,163.96
S$16949
  Bottom 0: 204.02,163.96 203.72,164.06
S$16950
  Bottom 0: 203.72,164.06 203.39,164.08
S$16951
  Bottom 0: 203.39,164.08 203.07,164.02
S$16952
  Bottom 0: 203.07,164.02 202.78,163.87
S$16953
  Bottom 0: 202.78,163.87 202.55,163.65
S$16954
  Bottom 0: 202.55,163.65 202.38,163.37
S$16955
  Bottom 0: 202.38,163.37 202.29,163.06
S$16956
  Bottom 0: 202.29,163.06 202.29,162.73
S$16957
  Bottom 0: 202.29,162.73 202.38,162.42
S$16958
  Bottom 0: 202.38,162.42 202.55,162.14
S$16959
  Bottom 0: 202.55,162.14 202.78,161.92
S$16960
  Bottom 0: 202.78,161.92 203.07,161.77
S$16961
  Bottom 0: 203.07,161.77 203.39,161.71
S$16962
  Bottom 0: 203.39,161.71 203.72,161.73
S$16963
  Bottom 0: 203.72,161.73 203.94,161.8
S$16964
  Bottom 0: 203.94,161.8 204.99,160.75
S$16965
  Bottom 0: 204.99,160.75 204.96,160.73
S$16966
  Bottom 0: 204.96,160.73 204.9,160.68
S$16967
  Bottom 0: 204.9,160.68 204.86,160.6
S$16968
  Bottom 0: 204.86,160.6 204.85,160.53
S$16969
  Bottom 0: 204.85,160.53 204.85,159.03
S$16970
  Bottom 0: 204.85,159.03 198.35,165.54
S$16971
  Bottom 0: 198.35,165.54 198.35,168.67
S$16972
  Bottom 0: 198.35,168.67 198.35,168.74
S$16973
  Bottom 0: 198.35,168.74 198.33,168.81
S$16974
  Bottom 0: 198.33,168.81 198.31,168.87
S$16975
  Bottom 0: 198.31,168.87 198.27,168.93
S$16976
  Bottom 0: 198.27,168.93 198.23,168.99
S$16977
  Bottom 0: 198.23,168.99 195.71,171.51
S$16978
  Bottom 0: 195.71,171.51 195.71,172.58
S$16979
  Bottom 0: 195.71,172.58 195.84,172.34
S$16980
  Bottom 0: 195.84,172.34 196.12,171.99
S$16981
  Bottom 0: 196.12,171.99 196.47,171.71
S$16982
  Bottom 0: 196.47,171.71 196.87,171.5
S$16983
  Bottom 0: 196.87,171.5 197.29,171.37
S$16984
  Bottom 0: 197.29,171.37 197.74,171.32
S$16985
  Bottom 0: 197.74,171.32 198.19,171.37
S$16986
  Bottom 0: 198.19,171.37 198.61,171.5
S$16987
  Bottom 0: 198.61,171.5 199.01,171.71
S$16988
  Bottom 0: 199.01,171.71 199.28,171.93
S$16989
  Bottom 0: 199.28,171.93 199.28,170.34
S$16990
  Bottom 0: 199.28,170.34 199.29,170.25
S$16991
  Bottom 0: 199.29,170.25 199.31,170.16
S$16992
  Bottom 0: 199.31,170.16 199.34,170.08
S$16993
  Bottom 0: 199.34,170.08 199.39,170
S$16994
  Bottom 0: 199.39,170 199.45,169.94
S$16995
  Bottom 0: 199.45,169.94 207.97,161.43
S$16996
  Bottom 0: 207.97,161.43 207.97,160.62
S$16997
  Bottom 0: 207.97,160.62 207.79,160.5
S$16998
  Bottom 0: 207.79,160.5 207.57,160.26
S$16999
  Bottom 0: 207.57,160.26 207.44,159.96
S$17000
  Bottom 0: 207.44,159.96 207.39,159.64
S$17001
  Bottom 0: 207.39,159.64 207.44,159.32
S$17002
  Bottom 0: 207.44,159.32 207.57,159.02
S$17003
  Bottom 0: 207.57,159.02 207.78,158.79
S$17004
  Bottom 0: 207.78,158.79 207.14,158.79
S$17005
  Bottom 0: 201.49,164.08 201.81,164.1
S$17006
  Bottom 0: 201.81,164.1 202.12,164.21
S$17007
  Bottom 0: 202.12,164.21 202.38,164.39
S$17008
  Bottom 0: 202.38,164.39 202.59,164.65
S$17009
  Bottom 0: 202.59,164.65 202.72,164.95
S$17010
  Bottom 0: 202.72,164.95 202.76,165.27
S$17011
  Bottom 0: 202.76,165.27 202.72,165.59
S$17012
  Bottom 0: 202.72,165.59 202.59,165.89
S$17013
  Bottom 0: 202.59,165.89 202.38,166.14
S$17014
  Bottom 0: 202.38,166.14 202.12,166.33
S$17015
  Bottom 0: 202.12,166.33 201.81,166.44
S$17016
  Bottom 0: 201.81,166.44 201.49,166.46
S$17017
  Bottom 0: 201.49,166.46 201.17,166.39
S$17018
  Bottom 0: 201.17,166.39 200.88,166.24
S$17019
  Bottom 0: 200.88,166.24 200.65,166.02
S$17020
  Bottom 0: 200.65,166.02 200.47,165.75
S$17021
  Bottom 0: 200.47,165.75 200.39,165.43
S$17022
  Bottom 0: 200.39,165.43 200.39,165.1
S$17023
  Bottom 0: 200.39,165.1 200.47,164.79
S$17024
  Bottom 0: 200.47,164.79 200.65,164.52
S$17025
  Bottom 0: 200.65,164.52 200.88,164.29
S$17026
  Bottom 0: 200.88,164.29 201.17,164.15
S$17027
  Bottom 0: 201.17,164.15 201.49,164.08
S$17028
  Bottom 0: 149.99,159.04 149.99,160.53
S$17029
  Bottom 0: 149.99,160.53 149.98,160.6
S$17030
  Bottom 0: 149.98,160.6 149.93,160.68
S$17031
  Bottom 0: 149.93,160.68 149.88,160.73
S$17032
  Bottom 0: 149.88,160.73 149.81,160.77
S$17033
  Bottom 0: 149.81,160.77 149.73,160.78
S$17034
  Bottom 0: 149.73,160.78 149.29,160.78
S$17035
  Bottom 0: 149.29,160.78 149.29,160.91
S$17036
  Bottom 0: 149.29,160.91 149.22,161.13
S$17037
  Bottom 0: 149.22,161.13 149.06,161.29
S$17038
  Bottom 0: 149.06,161.29 148.84,161.35
S$17039
  Bottom 0: 148.84,161.35 148.49,161.35
S$17040
  Bottom 0: 148.49,161.35 147.41,162.44
S$17041
  Bottom 0: 147.41,162.44 147.47,162.57
S$17042
  Bottom 0: 147.47,162.57 147.51,162.89
S$17043
  Bottom 0: 147.51,162.89 147.47,163.22
S$17044
  Bottom 0: 147.47,163.22 147.34,163.51
S$17045
  Bottom 0: 147.34,163.51 147.13,163.77
S$17046
  Bottom 0: 147.13,163.77 147.09,163.8
S$17047
  Bottom 0: 147.09,163.8 148.82,163.8
S$17048
  Bottom 0: 148.82,163.8 152.09,160.53
S$17049
  Bottom 0: 152.09,160.53 151.86,160.68
S$17050
  Bottom 0: 151.86,160.68 151.55,160.77
S$17051
  Bottom 0: 151.55,160.77 151.22,160.77
S$17052
  Bottom 0: 151.22,160.77 150.91,160.68
S$17053
  Bottom 0: 150.91,160.68 150.63,160.5
S$17054
  Bottom 0: 150.63,160.5 150.42,160.26
S$17055
  Bottom 0: 150.42,160.26 150.28,159.96
S$17056
  Bottom 0: 150.28,159.96 150.24,159.64
S$17057
  Bottom 0: 150.24,159.64 150.28,159.34
S$17058
  Bottom 0: 150.28,159.34 149.99,159.04
S$17059
  Bottom 0: 316.53,160.28 316.53,160.51
S$17060
  Bottom 0: 316.53,160.51 316.52,160.59
S$17061
  Bottom 0: 316.52,160.59 316.48,160.66
S$17062
  Bottom 0: 316.48,160.66 316.42,160.72
S$17063
  Bottom 0: 316.42,160.72 316.35,160.76
S$17064
  Bottom 0: 316.35,160.76 316.28,160.77
S$17065
  Bottom 0: 316.28,160.77 315.2,160.77
S$17066
  Bottom 0: 315.2,160.77 315.2,160.89
S$17067
  Bottom 0: 315.2,160.89 315.18,160.95
S$17068
  Bottom 0: 315.18,160.95 315.18,161.01
S$17069
  Bottom 0: 315.18,161.01 315.15,161.07
S$17070
  Bottom 0: 315.15,161.07 315.14,161.12
S$17071
  Bottom 0: 315.14,161.12 315.11,161.15
S$17072
  Bottom 0: 315.11,161.15 315.07,161.21
S$17073
  Bottom 0: 315.07,161.21 314.02,162.25
S$17074
  Bottom 0: 314.02,162.25 314.05,162.28
S$17075
  Bottom 0: 314.05,162.28 314.17,162.57
S$17076
  Bottom 0: 314.17,162.57 314.22,162.89
S$17077
  Bottom 0: 314.22,162.89 314.17,163.22
S$17078
  Bottom 0: 314.17,163.22 314.05,163.51
S$17079
  Bottom 0: 314.05,163.51 313.84,163.77
S$17080
  Bottom 0: 313.84,163.77 313.57,163.96
S$17081
  Bottom 0: 313.57,163.96 313.27,164.06
S$17082
  Bottom 0: 313.27,164.06 312.98,164.08
S$17083
  Bottom 0: 312.98,164.08 313.27,164.1
S$17084
  Bottom 0: 313.27,164.1 313.57,164.21
S$17085
  Bottom 0: 313.57,164.21 313.84,164.39
S$17086
  Bottom 0: 313.84,164.39 314.05,164.65
S$17087
  Bottom 0: 314.05,164.65 314.17,164.95
S$17088
  Bottom 0: 314.17,164.95 314.22,165.27
S$17089
  Bottom 0: 314.22,165.27 314.17,165.59
S$17090
  Bottom 0: 314.17,165.59 314.05,165.89
S$17091
  Bottom 0: 314.05,165.89 313.84,166.14
S$17092
  Bottom 0: 313.84,166.14 313.57,166.33
S$17093
  Bottom 0: 313.57,166.33 313.27,166.44
S$17094
  Bottom 0: 313.27,166.44 312.94,166.46
S$17095
  Bottom 0: 312.94,166.46 312.62,166.39
S$17096
  Bottom 0: 312.62,166.39 312.56,166.36
S$17097
  Bottom 0: 312.56,166.36 312.41,166.51
S$17098
  Bottom 0: 312.41,166.51 312.41,167.63
S$17099
  Bottom 0: 312.41,167.63 312.6,167.44
S$17100
  Bottom 0: 312.6,167.44 312.89,167.25
S$17101
  Bottom 0: 312.89,167.25 313.22,167.14
S$17102
  Bottom 0: 313.22,167.14 313.57,167.12
S$17103
  Bottom 0: 313.57,167.12 313.88,167.18
S$17104
  Bottom 0: 313.88,167.18 313.99,167.14
S$17105
  Bottom 0: 313.99,167.14 314.33,167.12
S$17106
  Bottom 0: 314.33,167.12 314.68,167.18
S$17107
  Bottom 0: 314.68,167.18 315,167.34
S$17108
  Bottom 0: 315,167.34 315.26,167.56
S$17109
  Bottom 0: 315.26,167.56 315.47,167.84
S$17110
  Bottom 0: 315.47,167.84 315.6,168.17
S$17111
  Bottom 0: 315.6,168.17 315.65,168.51
S$17112
  Bottom 0: 315.65,168.51 315.6,168.86
S$17113
  Bottom 0: 315.6,168.86 315.47,169.18
S$17114
  Bottom 0: 315.47,169.18 315.26,169.47
S$17115
  Bottom 0: 315.26,169.47 315,169.69
S$17116
  Bottom 0: 315,169.69 314.68,169.84
S$17117
  Bottom 0: 314.68,169.84 314.33,169.91
S$17118
  Bottom 0: 314.33,169.91 313.99,169.88
S$17119
  Bottom 0: 313.99,169.88 313.88,169.85
S$17120
  Bottom 0: 313.88,169.85 313.57,169.91
S$17121
  Bottom 0: 313.57,169.91 313.22,169.88
S$17122
  Bottom 0: 313.22,169.88 312.89,169.78
S$17123
  Bottom 0: 312.89,169.78 312.6,169.59
S$17124
  Bottom 0: 312.6,169.59 312.41,169.39
S$17125
  Bottom 0: 312.41,169.39 312.41,174.44
S$17126
  Bottom 0: 312.41,174.44 314.15,176.17
S$17127
  Bottom 0: 314.15,176.17 313,175.02
S$17128
  Bottom 0: 313,175.02 312.94,174.96
S$17129
  Bottom 0: 312.94,174.96 312.89,174.88
S$17130
  Bottom 0: 312.89,174.88 312.86,174.8
S$17131
  Bottom 0: 312.86,174.8 312.84,174.71
S$17132
  Bottom 0: 312.84,174.71 312.83,174.62
S$17133
  Bottom 0: 312.83,174.62 312.83,172.6
S$17134
  Bottom 0: 312.83,172.6 312.84,172.51
S$17135
  Bottom 0: 312.84,172.51 312.86,172.42
S$17136
  Bottom 0: 312.86,172.42 312.89,172.34
S$17137
  Bottom 0: 312.89,172.34 312.94,172.26
S$17138
  Bottom 0: 312.94,172.26 313,172.2
S$17139
  Bottom 0: 313,172.2 317.49,167.71
S$17140
  Bottom 0: 317.49,167.71 317.49,160.61
S$17141
  Bottom 0: 317.49,160.61 317.37,160.63
S$17142
  Bottom 0: 317.37,160.63 317.07,160.61
S$17143
  Bottom 0: 317.07,160.61 316.79,160.5
S$17144
  Bottom 0: 316.79,160.5 316.55,160.31
S$17145
  Bottom 0: 316.55,160.31 316.53,160.28
S$17146
  Bottom 0: 318.89,160.39 318.81,160.49
S$17147
  Bottom 0: 318.81,160.49 318.63,160.6
S$17148
  Bottom 0: 318.63,160.6 318.63,167.94
S$17149
  Bottom 0: 318.63,167.94 318.62,168.03
S$17150
  Bottom 0: 318.62,168.03 318.6,168.12
S$17151
  Bottom 0: 318.6,168.12 318.57,168.2
S$17152
  Bottom 0: 318.57,168.2 318.52,168.28
S$17153
  Bottom 0: 318.52,168.28 318.46,168.34
S$17154
  Bottom 0: 318.46,168.34 315.39,171.41
S$17155
  Bottom 0: 315.39,171.41 315.57,171.35
S$17156
  Bottom 0: 315.57,171.35 316.02,171.31
S$17157
  Bottom 0: 316.02,171.31 316.4,171.35
S$17158
  Bottom 0: 316.4,171.35 316.78,171.31
S$17159
  Bottom 0: 316.78,171.31 317.23,171.35
S$17160
  Bottom 0: 317.23,171.35 317.65,171.48
S$17161
  Bottom 0: 317.65,171.48 318.05,171.69
S$17162
  Bottom 0: 318.05,171.69 318.4,171.98
S$17163
  Bottom 0: 318.4,171.98 318.68,172.32
S$17164
  Bottom 0: 318.68,172.32 318.9,172.72
S$17165
  Bottom 0: 318.9,172.72 319.02,173.15
S$17166
  Bottom 0: 319.02,173.15 319.07,173.59
S$17167
  Bottom 0: 319.07,173.59 319.02,174.04
S$17168
  Bottom 0: 319.02,174.04 318.98,174.19
S$17169
  Bottom 0: 318.98,174.19 320.73,172.44
S$17170
  Bottom 0: 320.73,172.44 320.69,172.45
S$17171
  Bottom 0: 320.69,172.45 320.33,172.43
S$17172
  Bottom 0: 320.33,172.43 320.23,172.39
S$17173
  Bottom 0: 320.23,172.39 319.92,172.45
S$17174
  Bottom 0: 319.92,172.45 319.57,172.43
S$17175
  Bottom 0: 319.57,172.43 319.24,172.32
S$17176
  Bottom 0: 319.24,172.32 318.95,172.13
S$17177
  Bottom 0: 318.95,172.13 318.71,171.88
S$17178
  Bottom 0: 318.71,171.88 318.54,171.57
S$17179
  Bottom 0: 318.54,171.57 318.45,171.23
S$17180
  Bottom 0: 318.45,171.23 318.45,170.88
S$17181
  Bottom 0: 318.45,170.88 318.54,170.54
S$17182
  Bottom 0: 318.54,170.54 318.71,170.23
S$17183
  Bottom 0: 318.71,170.23 318.89,170.04
S$17184
  Bottom 0: 318.89,170.04 318.89,160.39
S$17185
  Bottom 0: 194.58,163.01 193.35,164.25
S$17186
  Bottom 0: 193.35,164.25 193.55,164.15
S$17187
  Bottom 0: 193.55,164.15 193.87,164.08
S$17188
  Bottom 0: 193.87,164.08 194.19,164.1
S$17189
  Bottom 0: 194.19,164.1 194.5,164.21
S$17190
  Bottom 0: 194.5,164.21 194.76,164.39
S$17191
  Bottom 0: 194.76,164.39 194.97,164.65
S$17192
  Bottom 0: 194.97,164.65 195.09,164.95
S$17193
  Bottom 0: 195.09,164.95 195.14,165.27
S$17194
  Bottom 0: 195.14,165.27 195.09,165.59
S$17195
  Bottom 0: 195.09,165.59 194.97,165.89
S$17196
  Bottom 0: 194.97,165.89 194.76,166.14
S$17197
  Bottom 0: 194.76,166.14 194.5,166.33
S$17198
  Bottom 0: 194.5,166.33 194.19,166.44
S$17199
  Bottom 0: 194.19,166.44 194,166.44
S$17200
  Bottom 0: 194,166.44 194,167.84
S$17201
  Bottom 0: 194,167.84 194.07,167.71
S$17202
  Bottom 0: 194.07,167.71 194.31,167.45
S$17203
  Bottom 0: 194.31,167.45 194.6,167.26
S$17204
  Bottom 0: 194.6,167.26 194.94,167.16
S$17205
  Bottom 0: 194.94,167.16 195.28,167.14
S$17206
  Bottom 0: 195.28,167.14 195.63,167.2
S$17207
  Bottom 0: 195.63,167.2 195.95,167.35
S$17208
  Bottom 0: 195.95,167.35 196.22,167.57
S$17209
  Bottom 0: 196.22,167.57 196.42,167.86
S$17210
  Bottom 0: 196.42,167.86 196.55,168.18
S$17211
  Bottom 0: 196.55,168.18 196.6,168.53
S$17212
  Bottom 0: 196.6,168.53 196.55,168.87
S$17213
  Bottom 0: 196.55,168.87 196.42,169.2
S$17214
  Bottom 0: 196.42,169.2 196.22,169.48
S$17215
  Bottom 0: 196.22,169.48 195.95,169.71
S$17216
  Bottom 0: 195.95,169.71 195.63,169.86
S$17217
  Bottom 0: 195.63,169.86 195.28,169.92
S$17218
  Bottom 0: 195.28,169.92 194.94,169.9
S$17219
  Bottom 0: 194.94,169.9 194.6,169.79
S$17220
  Bottom 0: 194.6,169.79 194.31,169.61
S$17221
  Bottom 0: 194.31,169.61 194.07,169.35
S$17222
  Bottom 0: 194.07,169.35 194,169.22
S$17223
  Bottom 0: 194,169.22 194,174.32
S$17224
  Bottom 0: 194,174.32 196.78,177.1
S$17225
  Bottom 0: 196.78,177.1 196.81,177.16
S$17226
  Bottom 0: 196.81,177.16 196.85,177.2
S$17227
  Bottom 0: 196.85,177.2 196.87,177.25
S$17228
  Bottom 0: 196.87,177.25 196.9,177.3
S$17229
  Bottom 0: 196.9,177.3 196.9,177.36
S$17230
  Bottom 0: 196.9,177.36 196.91,177.42
S$17231
  Bottom 0: 196.91,177.42 196.91,177.55
S$17232
  Bottom 0: 196.91,177.55 197.28,177.55
S$17233
  Bottom 0: 197.28,177.55 197.28,177.18
S$17234
  Bottom 0: 197.28,177.18 194.95,174.85
S$17235
  Bottom 0: 194.95,174.85 194.91,174.79
S$17236
  Bottom 0: 194.91,174.79 194.87,174.73
S$17237
  Bottom 0: 194.87,174.73 194.84,174.67
S$17238
  Bottom 0: 194.84,174.67 194.83,174.6
S$17239
  Bottom 0: 194.83,174.6 194.82,174.53
S$17240
  Bottom 0: 194.82,174.53 194.82,171.32
S$17241
  Bottom 0: 194.82,171.32 194.83,171.25
S$17242
  Bottom 0: 194.83,171.25 194.84,171.18
S$17243
  Bottom 0: 194.84,171.18 194.87,171.12
S$17244
  Bottom 0: 194.87,171.12 194.91,171.06
S$17245
  Bottom 0: 194.91,171.06 194.95,171
S$17246
  Bottom 0: 194.95,171 197.47,168.48
S$17247
  Bottom 0: 197.47,168.48 197.47,165.35
S$17248
  Bottom 0: 197.47,165.35 197.47,165.28
S$17249
  Bottom 0: 197.47,165.28 197.49,165.22
S$17250
  Bottom 0: 197.49,165.22 197.51,165.16
S$17251
  Bottom 0: 197.51,165.16 197.56,165.09
S$17252
  Bottom 0: 197.56,165.09 197.6,165.04
S$17253
  Bottom 0: 197.6,165.04 199.62,163.01
S$17254
  Bottom 0: 199.62,163.01 194.58,163.01
S$17255
  Bottom 0: 78.77,163.46 78.75,163.51
S$17256
  Bottom 0: 78.75,163.51 78.54,163.77
S$17257
  Bottom 0: 78.54,163.77 78.28,163.96
S$17258
  Bottom 0: 78.28,163.96 77.97,164.06
S$17259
